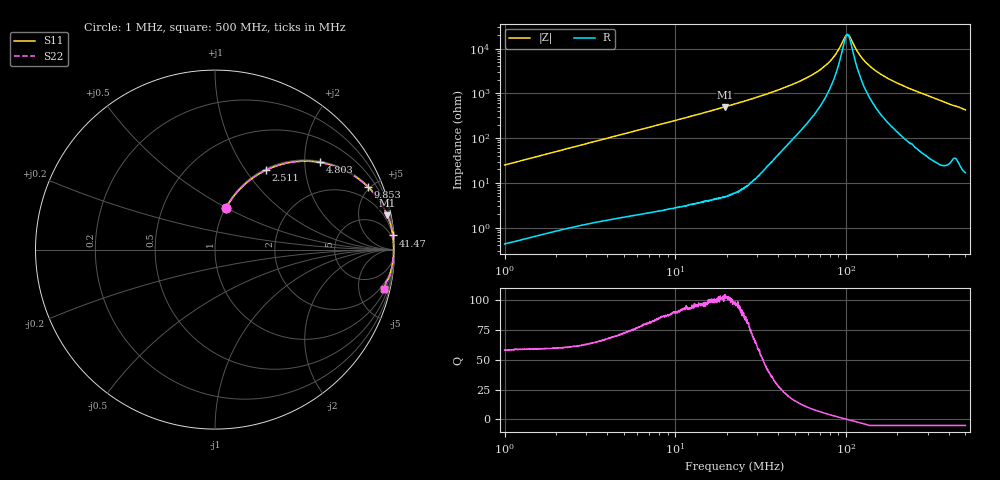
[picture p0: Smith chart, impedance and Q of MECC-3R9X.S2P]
!s-Parameter Generated by FASTRON Sdn. Bhd.
!FASTRON P/N : MECC-3R9X
!Keysight Technologies,E4991B,MY54100416,A.01.15
!Date: Thu Apr 02 09:22:27 2026
!Version  : Rev00 Thu Apr 02 09:22:27 2026
!Data & Calibration Information:
!PortZ  Port1:50+j0  Port2:50+j0
!When reading, reference impedance value at option line is always used.
! Remarks : This data is being provided solely for informational purposes.
!Freq	S11	S21	S12	S22
# Hz S dB R 50
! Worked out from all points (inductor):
!   1601 points, 1 MHz to 500 MHz, reference 50 ohm
!   read as one part in series: L = 3.98 uH near 1.032 MHz
!   highest Q = 102 at 19.52 MHz (marker M1), where L = 4.06 uH
!   self-resonance near 101.7 MHz
!   S11 on the Smith chart (normalised r, x): 1 MHz: 1.01, +0.50; 2.511 MHz: 1.02, +1.25; 4.803 MHz: 1.03, +2.37; 9.853 MHz: 1.05, +4.88; 41.47 MHz: 2, +25; 500 MHz: 1.34, -8.53
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1000000  -12.33 75.0  -0.30 -14.0  -0.30 -14.0  -12.33 75.0
1618714  -8.58 67.2  -0.71 -21.8  -0.71 -21.8  -8.58 67.2
2510643  -5.60 57.4  -1.49 -31.7  -1.49 -31.7  -5.60 57.4
2820919  -4.90 54.4  -1.80 -34.7  -1.80 -34.7  -4.90 54.4
4802749  -2.39 39.8  -3.88 -49.4  -3.88 -49.4  -2.39 39.8
7957584  -1.04 26.8  -6.92 -62.5  -6.92 -62.5  -1.04 26.8
9852770  -0.71 22.2  -8.46 -67.2  -8.46 -67.2  -0.71 22.2
1.951844e7  -0.19 11.3  -14.14 -78.1  -14.14 -78.1  -0.19 11.3
2.236068e7  -0.14 9.8  -15.40 -79.6  -15.40 -79.6  -0.14 9.8
4.146629e7  -0.05 4.6  -22.00 -83.2  -22.00 -83.2  -0.05 4.6
6.307767e7  -0.04 2.2  -28.23 -81.3  -28.23 -81.3  -0.04 2.2
8.150948e7  -0.04 1.0  -34.85 -73.8  -34.85 -73.8  -0.04 1.0
8.878078e7  -0.04 0.6  -38.59 -65.7  -38.59 -65.7  -0.04 0.6
9.859709e7  -0.04 0.1  -45.26 -28.2  -45.26 -28.2  -0.04 0.1
1.021047e8  -0.04 -0.0  -46.36 1.3  -46.36 1.3  -0.04 -0.0
1.057371e8  -0.04 -0.2  -45.05 30.5  -45.05 30.5  -0.04 -0.2
1.192669e8  -0.04 -0.7  -37.58 68.0  -37.58 68.0  -0.04 -0.7
1.304121e8  -0.04 -1.1  -33.93 75.1  -33.93 75.1  -0.04 -1.1
1.488233e8  -0.05 -1.8  -30.17 79.5  -30.17 79.5  -0.05 -1.8
1.77937e8  -0.05 -2.7  -26.53 81.6  -26.53 81.6  -0.05 -2.7
2.613756e8  -0.08 -5.2  -20.87 81.8  -20.87 81.8  -0.08 -5.2
5e8  -0.31 -13.1  -12.92 74.7  -12.92 74.7  -0.31 -13.1
